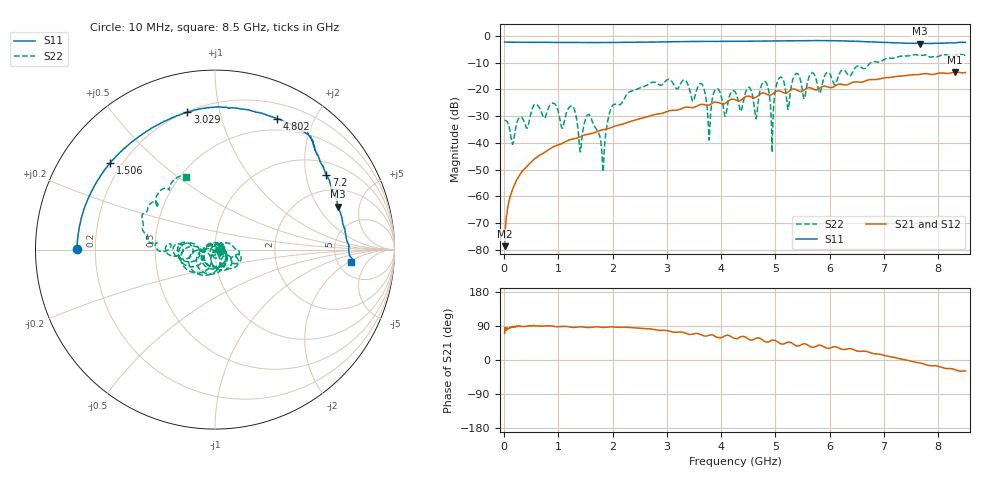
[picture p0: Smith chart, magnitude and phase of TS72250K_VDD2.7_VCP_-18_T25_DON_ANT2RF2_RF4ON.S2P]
!Agilent Technologies,E5071C,MY46417908,A.11.23
!Date: Thu Oct 03 13:34:00 2019
!Data & Calibration Information:
!Freq	S11:SOLT2(ON)	S21:SOLT2(ON)	S12:SOLT2(ON)	S22:SOLT2(ON)
!PortZ  Port1:50+j0  Port2:50+j0
!Above PortZ is port z conversion or system Z0 setting when saving the data.
!When reading, reference impedance value at option line is always used.
# Hz S dB R 50
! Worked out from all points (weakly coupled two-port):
!   1601 points, 10 MHz to 8.5 GHz, reference 50 ohm
!   highest |S21| = -13.51 dB at 8.314 GHz (marker M1); lowest = -78.7 dB at 10 MHz (marker M2)
!   lowest |S11| = -2.8 dB at 7.662 GHz (marker M3), VSWR 6.30, Z = 151 + j153 ohm
!   |S11| at or under -10 dB: nowhere
!   |S22| runs from -50.8 to -6.9 dB; largest |S21 - S12| = 0.0021
!   S11 on the Smith chart (normalised r, x): 10 MHz: 0.13, +0.00; 1.506 GHz: 0.16, +0.35; 3.029 GHz: 0.20, +0.80; 4.802 GHz: 0.36, +1.52; 7.2 GHz: 1.40, +2.62; 8.5 GHz: 6.67, -2.24
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1e7  -2.26 179.9  -78.70 69.9  -82.20 83.6  -31.67 -0.3
3.177625e8  -2.32 171.8  -51.16 89.1  -51.10 88.9  -30.40 22.6
1.246356e9  -2.39 147.4  -38.65 86.3  -38.66 86.3  -26.20 -75.3
1.426769e9  -2.41 142.5  -37.48 87.5  -37.50 87.2  -39.72 -53.3
1.506362e9  -2.41 140.4  -36.92 86.2  -36.90 85.9  -30.78 -88.2
1.819431e9  -2.42 131.9  -35.11 86.2  -35.09 86.1  -50.08 49.3
1.999844e9  -2.41 127.0  -34.04 87.6  -34.02 87.5  -25.99 48.1
2.843538e9  -2.22 105.4  -29.17 78.7  -29.12 78.6  -18.07 -18.4
3.029256e9  -2.15 101.4  -28.10 76.8  -28.05 76.9  -16.20 -21.0
3.639475e9  -2.01 89.5  -25.59 65.9  -25.57 66.0  -17.91 -64.8
3.777438e9  -2.00 86.6  -25.84 65.2  -25.85 65.4  -38.98 -77.8
4.255e9  -1.94 76.9  -23.84 56.5  -23.84 56.5  -20.84 -128.5
4.642356e9  -1.90 68.2  -22.95 57.4  -22.93 57.5  -31.01 75.0
4.801544e9  -1.85 64.6  -21.43 49.0  -21.39 49.1  -16.99 -116.4
4.939506e9  -1.83 62.0  -21.82 52.3  -21.82 52.5  -43.53 -115.2
5.072162e9  -1.77 59.2  -20.55 44.6  -20.48 44.8  -15.70 -122.8
5.671769e9  -1.65 51.5  -19.62 33.9  -19.63 34.1  -13.80 -167.9
7.088538e9  -2.42 36.8  -15.50 9.2  -15.53 9.1  -8.32 170.1
7.199969e9  -2.54 33.8  -15.22 6.6  -15.25 6.3  -8.18 167.5
7.661612e9  -2.78 19.3  -14.36 -7.8  -14.33 -7.9  -7.23 150.9
8.314281e9  -2.50 -2.1  -13.51 -25.7  -13.52 -25.8  -7.31 125.8
8.5e9  -2.35 -5.3  -13.65 -28.8  -13.72 -29.2  -7.24 112.1
